(* Logix 5000 AddOnInstructionDefinition export PRNG; software revision 30.00 *)

ADD_ON_INSTRUCTION D_SHR   (* revision 1.0 20170524, vendor Kenneth A. Fischer *)
// DINT bit shift right of the 32-bit argument Inp_A by Inp_B bits with paddding by zeros on the right
// Revision note:
// Rev1.0: 20170524 - Initial Release
VAR_IN_OUT
   Inp_A : DINT; {required}   // 64-bit Integer to be right circular rotated
END_VAR
VAR_INPUT
   Inp_B : INT; {required}   // Number of bits to shift
END_VAR
VAR_IN_OUT
   Out : DINT; {required}   // Result
END_VAR
VAR
   BSR_Cntrl : CONTROL := (LEN := 32);
   ONS : BOOL;
   Source_Bit : BOOL;
   Wrk_InpA : DINT[2];
END_VAR

ROUTINE Logic   (* ladder *)
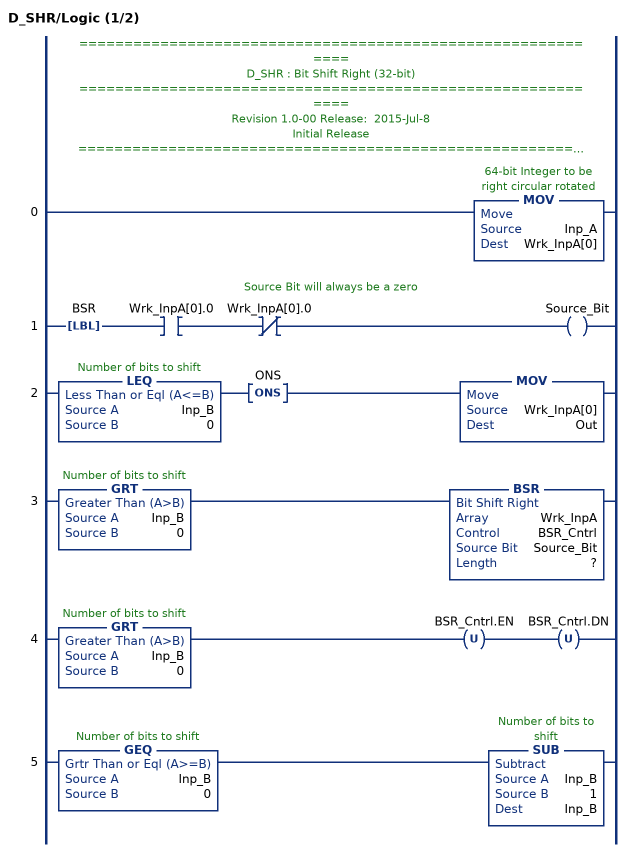
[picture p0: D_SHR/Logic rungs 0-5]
   // ============================================================
   // D_SHR : Bit Shift Right (32-bit)
   // ============================================================
   // Revision 1.0-00 Release:  2015-Jul-8
   // Initial Release
   // ============================================================
   // Performs a right bit shift of the 32-bit argument Inp_A by the
   // number of bits defined in the 16-bit argument Inp_B, with padding by zeros.
   0: MOV(Inp_A,Wrk_InpA[0]);
   // Source Bit will always be a zero
   1: LBL(BSR)XIC(Wrk_InpA[0].0)XIO(Wrk_InpA[0].0)OTE(Source_Bit);
   2: LEQ(Inp_B,0)ONS(ONS)MOV(Wrk_InpA[0],Out);
   3: GRT(Inp_B,0)BSR(Wrk_InpA,BSR_Cntrl,Source_Bit,?);
   4: GRT(Inp_B,0)OTU(BSR_Cntrl.EN)OTU(BSR_Cntrl.DN);
   5: GEQ(Inp_B,0)SUB(Inp_B,1,Inp_B);
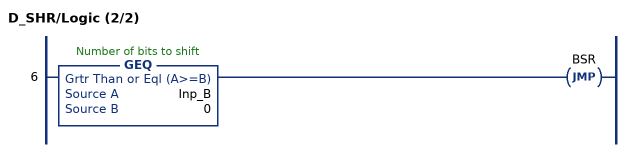
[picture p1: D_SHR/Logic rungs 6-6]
   6: GEQ(Inp_B,0)JMP(BSR);
END_ROUTINE
END_ADD_ON_INSTRUCTION

ADD_ON_INSTRUCTION D_SHL   (* revision 1.0 20170524, vendor Kenneth A. Fischer *)
// DINT bit shift left of the 32-bit argument Inp_A by Inp_B bits with paddding by zeros on the right
// Revision note:
// Rev1.0: 20170524 - Initial Release
VAR_IN_OUT
   Inp_A : DINT; {required}   // 64-bit Integer to be right circular rotated
END_VAR
VAR_INPUT
   Inp_B : INT; {required}   // Number of bits to shift
END_VAR
VAR_IN_OUT
   Out : DINT; {required}   // Result
END_VAR
VAR
   Wrk_InpA : DINT[2];
   Source_Bit : BOOL;
   ONS : BOOL;
   BSL_Cntrl : CONTROL := (LEN := 32);
END_VAR

ROUTINE Logic   (* ladder *)
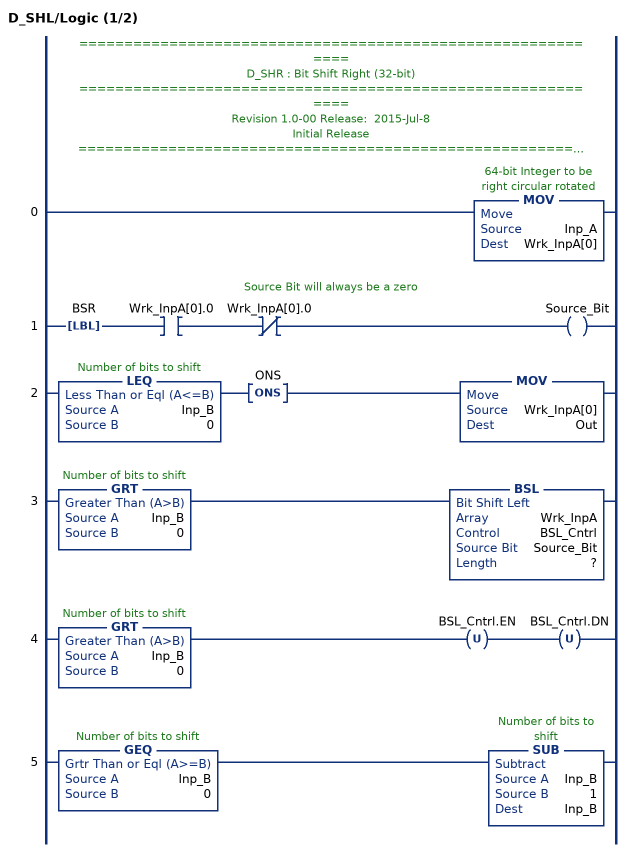
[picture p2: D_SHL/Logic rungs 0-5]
   // ============================================================
   // D_SHR : Bit Shift Right (32-bit)
   // ============================================================
   // Revision 1.0-00 Release:  2015-Jul-8
   // Initial Release
   // ============================================================
   // Performs a left bit shift of the 32-bit argument Inp_A by the
   // number of bits defined in the 16-bit argument Inp_B, with padding by zeros.
   0: MOV(Inp_A,Wrk_InpA[0]);
   // Source Bit will always be a zero
   1: LBL(BSR)XIC(Wrk_InpA[0].0)XIO(Wrk_InpA[0].0)OTE(Source_Bit);
   2: LEQ(Inp_B,0)ONS(ONS)MOV(Wrk_InpA[0],Out);
   3: GRT(Inp_B,0)BSL(Wrk_InpA,BSL_Cntrl,Source_Bit,?);
   4: GRT(Inp_B,0)OTU(BSL_Cntrl.EN)OTU(BSL_Cntrl.DN);
   5: GEQ(Inp_B,0)SUB(Inp_B,1,Inp_B);
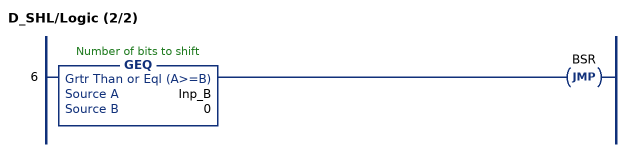
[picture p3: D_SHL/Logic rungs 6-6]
   6: GEQ(Inp_B,0)JMP(BSR);
END_ROUTINE
END_ADD_ON_INSTRUCTION

ADD_ON_INSTRUCTION B256_CtoE   (* revision 1.0 20170916, vendor Kenneth A. Fischer *)
// Convert 256-bit value using 22 12-bit pieces into 256-bit value using 32 8-bit pieces
// Revision note:
// Rev1.0: 20170916 - Initial Release
VAR_IN_OUT
   Inp_C : DINT[22]; {required}
   Out_E : DINT[32]; {required}
END_VAR
VAR
   i : INT;
   j : INT;
   TEMP1 : DINT;
   TEMP2 : DINT;
   D_SHL : D_SHL;
   D_SHR : D_SHR;
END_VAR

ROUTINE Logic   (* ladder *)
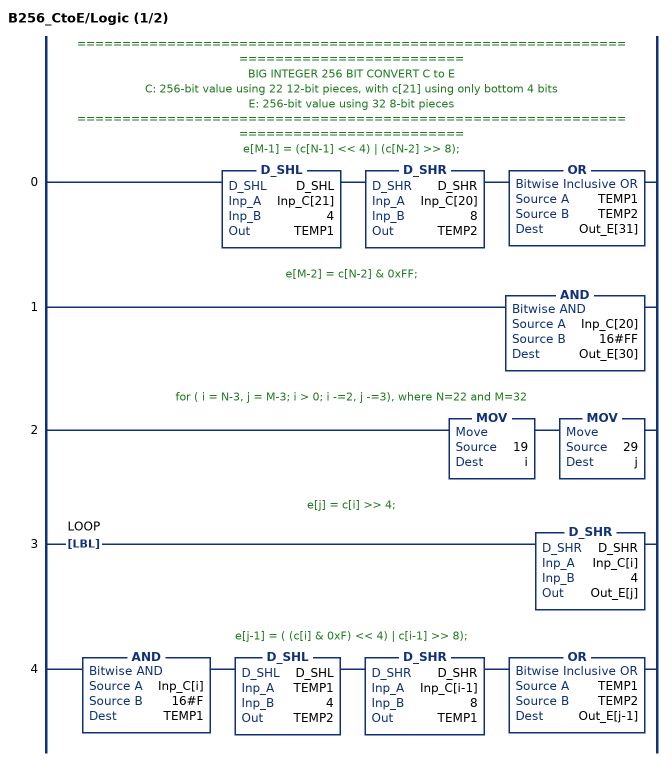
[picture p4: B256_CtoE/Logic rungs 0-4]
   // ======================================================================================
   // BIG INTEGER 256 BIT CONVERT C to E
   // C: 256-bit value using 22 12-bit pieces, with c[21] using only bottom 4 bits
   // E: 256-bit value using 32 8-bit pieces
   // ======================================================================================
   // e[M-1] = (c[N-1] << 4) | (c[N-2] >> 8);
   0: D_SHL(D_SHL,Inp_C[21],4,TEMP1)D_SHR(D_SHR,Inp_C[20],8,TEMP2)OR(TEMP1,TEMP2,Out_E[31]);
   // e[M-2] = c[N-2] & 0xFF;
   1: AND(Inp_C[20],16#FF,Out_E[30]);
   // for ( i = N-3, j = M-3; i > 0; i -=2, j -=3), where N=22 and M=32
   2: MOV(19,i)MOV(29,j);
   // e[j] = c[i] >> 4;
   3: LBL(LOOP)D_SHR(D_SHR,Inp_C[i],4,Out_E[j]);
   // e[j-1] = ( (c[i] & 0xF) << 4) | c[i-1] >> 8);
   4: AND(Inp_C[i],16#F,TEMP1)D_SHL(D_SHL,TEMP1,4,TEMP2)D_SHR(D_SHR,Inp_C[i-1],8,TEMP1)OR(TEMP1,TEMP2,Out_E[j-1]);
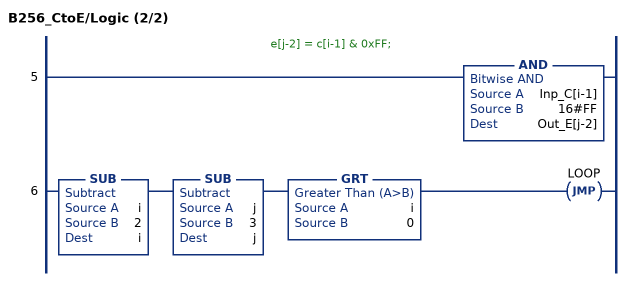
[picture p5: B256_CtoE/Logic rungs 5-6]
   // e[j-2] = c[i-1] & 0xFF;
   5: AND(Inp_C[i-1],16#FF,Out_E[j-2]);
   6: SUB(i,2,i)SUB(j,3,j)GRT(i,0)JMP(LOOP);
END_ROUTINE
END_ADD_ON_INSTRUCTION

ADD_ON_INSTRUCTION B256_CtoS   (* revision 1.0 20170916, vendor Kenneth A. Fischer *)
// Convert 256-bit value using 22 12-bit pieces into 64 hex big endian string characters
// Revision note:
// Rev1.0: 20170916 - Initial Release
VAR_IN_OUT
   Inp_C : DINT[22]; {required}
   Out_S : STRING; {required}
END_VAR
VAR
   byte : DINT[3];
   i : INT;
   j : INT;
   k : DINT;
   D_SHR : D_SHR;
END_VAR

ROUTINE Logic   (* ladder *)
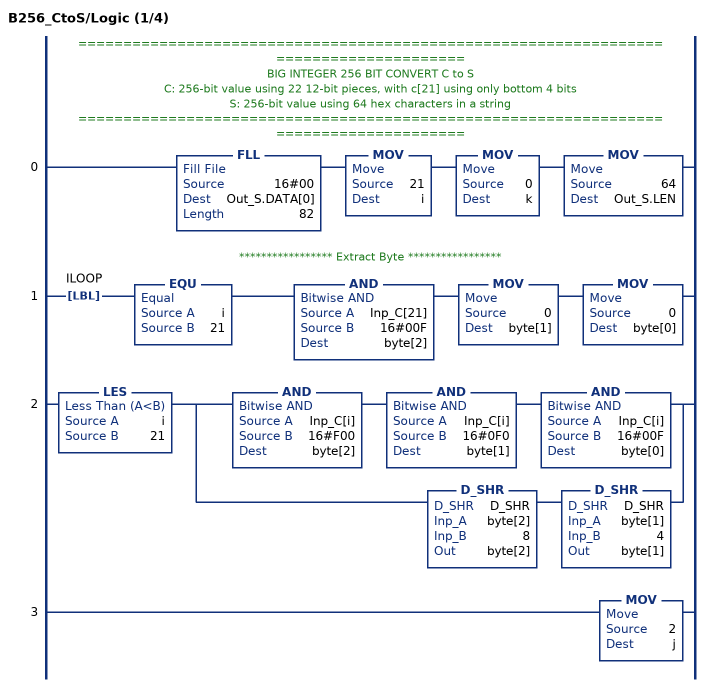
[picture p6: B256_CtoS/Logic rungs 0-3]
   // ======================================================================================
   // BIG INTEGER 256 BIT CONVERT C to S
   // C: 256-bit value using 22 12-bit pieces, with c[21] using only bottom 4 bits
   // S: 256-bit value using 64 hex characters in a string
   // ======================================================================================
   0: FLL(16#00,Out_S.DATA[0],82)MOV(21,i)MOV(0,k)MOV(64,Out_S.LEN);
   // ***************** Extract Byte *****************
   1: LBL(ILOOP)EQU(i,21)AND(Inp_C[21],16#00F,byte[2])MOV(0,byte[1])MOV(0,byte[0]);
   2: LES(i,21)[AND(Inp_C[i],16#F00,byte[2]) AND(Inp_C[i],16#0F0,byte[1]) AND(Inp_C[i],16#00F,byte[0]) ,D_SHR(D_SHR,byte[2],8,byte[2]) D_SHR(D_SHR,byte[1],4,byte[1]) ];
   3: MOV(2,j);
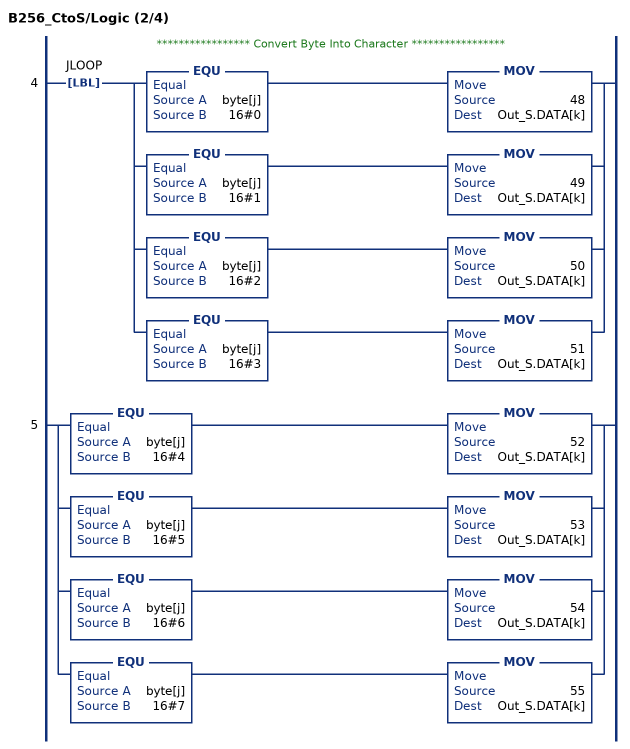
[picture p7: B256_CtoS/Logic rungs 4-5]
   // ***************** Convert Byte Into Character *****************
   4: LBL(JLOOP)[EQU(byte[j],16#0) MOV(48,Out_S.DATA[k]) ,EQU(byte[j],16#1) MOV(49,Out_S.DATA[k]) ,EQU(byte[j],16#2) MOV(50,Out_S.DATA[k]) ,EQU(byte[j],16#3) MOV(51,Out_S.DATA[k]) ];
   5: [EQU(byte[j],16#4) MOV(52,Out_S.DATA[k]) ,EQU(byte[j],16#5) MOV(53,Out_S.DATA[k]) ,EQU(byte[j],16#6) MOV(54,Out_S.DATA[k]) ,EQU(byte[j],16#7) MOV(55,Out_S.DATA[k]) ];
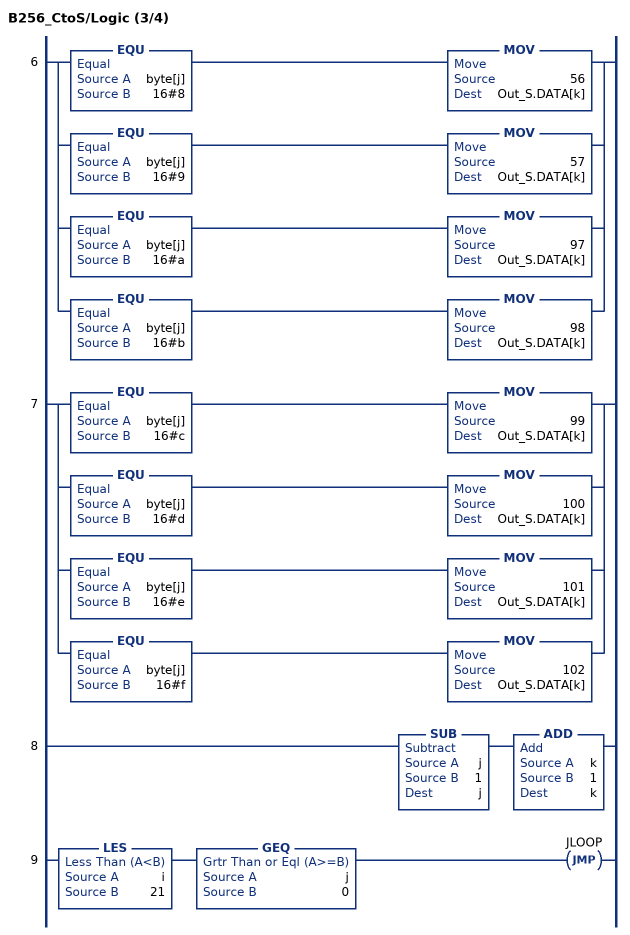
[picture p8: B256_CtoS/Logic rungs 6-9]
   6: [EQU(byte[j],16#8) MOV(56,Out_S.DATA[k]) ,EQU(byte[j],16#9) MOV(57,Out_S.DATA[k]) ,EQU(byte[j],16#a) MOV(97,Out_S.DATA[k]) ,EQU(byte[j],16#b) MOV(98,Out_S.DATA[k]) ];
   7: [EQU(byte[j],16#c) MOV(99,Out_S.DATA[k]) ,EQU(byte[j],16#d) MOV(100,Out_S.DATA[k]) ,EQU(byte[j],16#e) MOV(101,Out_S.DATA[k]) ,EQU(byte[j],16#f) MOV(102,Out_S.DATA[k]) ];
   8: SUB(j,1,j)ADD(k,1,k);
   9: LES(i,21)GEQ(j,0)JMP(JLOOP);
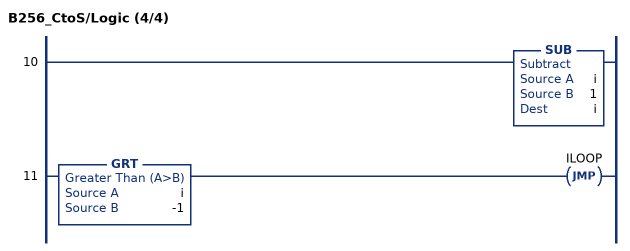
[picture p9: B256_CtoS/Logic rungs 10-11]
   10: SUB(i,1,i);
   11: GRT(i,-1)JMP(ILOOP);
END_ROUTINE
END_ADD_ON_INSTRUCTION

ADD_ON_INSTRUCTION B256_EtoL   (* revision 1.0 20170916, vendor Kenneth A. Fischer *)
// Convert 256-bit value using 32 8-bit pieces into 256-bit value using 4 64-bit pieces
// Revision note:
// Rev1.0: 20170916 - Initial Release
VAR_IN_OUT
   Inp_E : DINT[32]; {required}
   Out_L : LINT[4]; {required}
END_VAR
VAR
   D_SHL : D_SHL;
   Wrk_Out : DINT[2];
   i : INT;
   j : INT;
   TEMP : DINT;
END_VAR

ROUTINE Logic   (* ladder *)
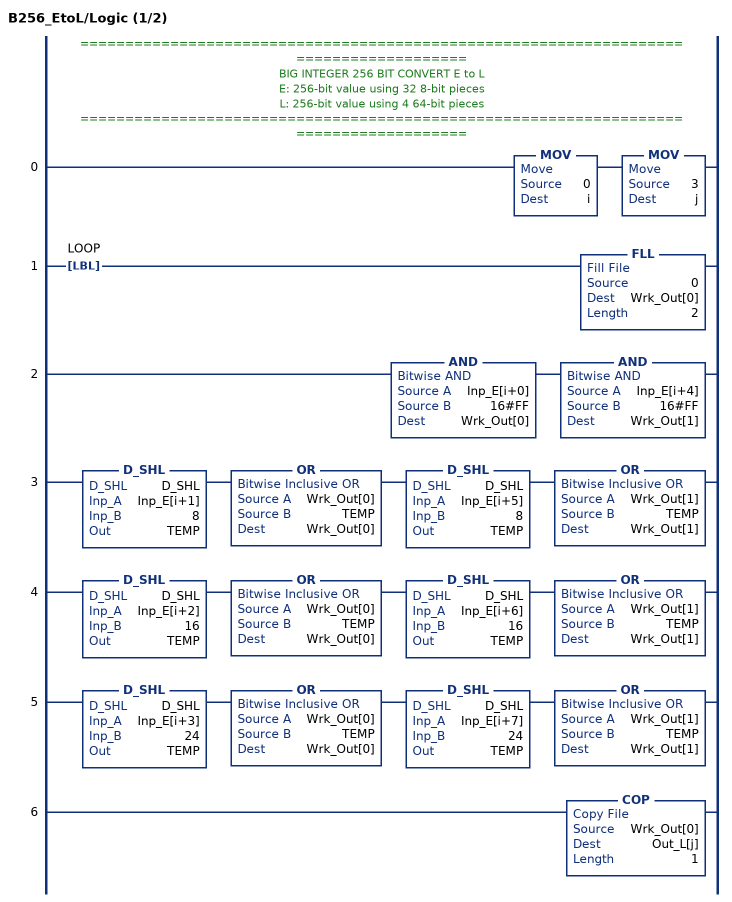
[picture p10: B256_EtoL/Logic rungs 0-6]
   // ======================================================================================
   // BIG INTEGER 256 BIT CONVERT E to L
   // E: 256-bit value using 32 8-bit pieces
   // L: 256-bit value using 4 64-bit pieces
   // ======================================================================================
   0: MOV(0,i)MOV(3,j);
   1: LBL(LOOP)FLL(0,Wrk_Out[0],2);
   2: AND(Inp_E[i+0],16#FF,Wrk_Out[0])AND(Inp_E[i+4],16#FF,Wrk_Out[1]);
   3: D_SHL(D_SHL,Inp_E[i+1],8,TEMP)OR(Wrk_Out[0],TEMP,Wrk_Out[0])D_SHL(D_SHL,Inp_E[i+5],8,TEMP)OR(Wrk_Out[1],TEMP,Wrk_Out[1]);
   4: D_SHL(D_SHL,Inp_E[i+2],16,TEMP)OR(Wrk_Out[0],TEMP,Wrk_Out[0])D_SHL(D_SHL,Inp_E[i+6],16,TEMP)OR(Wrk_Out[1],TEMP,Wrk_Out[1]);
   5: D_SHL(D_SHL,Inp_E[i+3],24,TEMP)OR(Wrk_Out[0],TEMP,Wrk_Out[0])D_SHL(D_SHL,Inp_E[i+7],24,TEMP)OR(Wrk_Out[1],TEMP,Wrk_Out[1]);
   6: COP(Wrk_Out[0],Out_L[j],1);
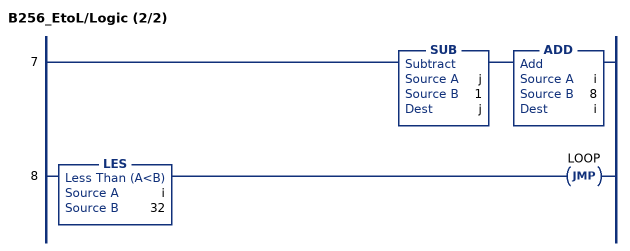
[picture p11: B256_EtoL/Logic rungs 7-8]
   7: SUB(j,1,j)ADD(i,8,i);
   8: LES(i,32)JMP(LOOP);
END_ROUTINE
END_ADD_ON_INSTRUCTION

ADD_ON_INSTRUCTION B256_StoC   (* revision 1.0 20170916, vendor Kenneth A. Fischer *)
// Convert 256-bit value using 64 hex string characters into 256-bit value using 22 12-bit pieces
// Revision note:
// Rev1.0: 20170916 - Initial Release
VAR_IN_OUT
   Inp_S : STRING; {required}
   Out_C : DINT[22]; {required}
END_VAR
VAR
   byte : DINT[3];
   D_SHL : D_SHL;
   i : INT;
   j : INT;
   k : DINT;
   temp : DINT;
END_VAR

ROUTINE Logic   (* ladder *)
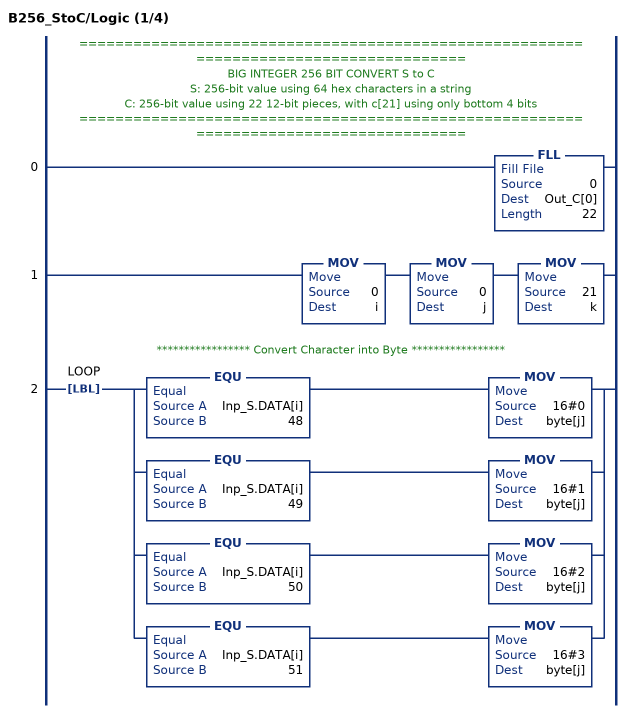
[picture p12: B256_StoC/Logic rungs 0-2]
   // ======================================================================================
   // BIG INTEGER 256 BIT CONVERT S to C
   // S: 256-bit value using 64 hex characters in a string
   // C: 256-bit value using 22 12-bit pieces, with c[21] using only bottom 4 bits
   // ======================================================================================
   0: FLL(0,Out_C[0],22);
   1: MOV(0,i)MOV(0,j)MOV(21,k);
   // ***************** Convert Character into Byte *****************
   2: LBL(LOOP)[EQU(Inp_S.DATA[i],48) MOV(16#0,byte[j]) ,EQU(Inp_S.DATA[i],49) MOV(16#1,byte[j]) ,EQU(Inp_S.DATA[i],50) MOV(16#2,byte[j]) ,EQU(Inp_S.DATA[i],51) MOV(16#3,byte[j]) ];
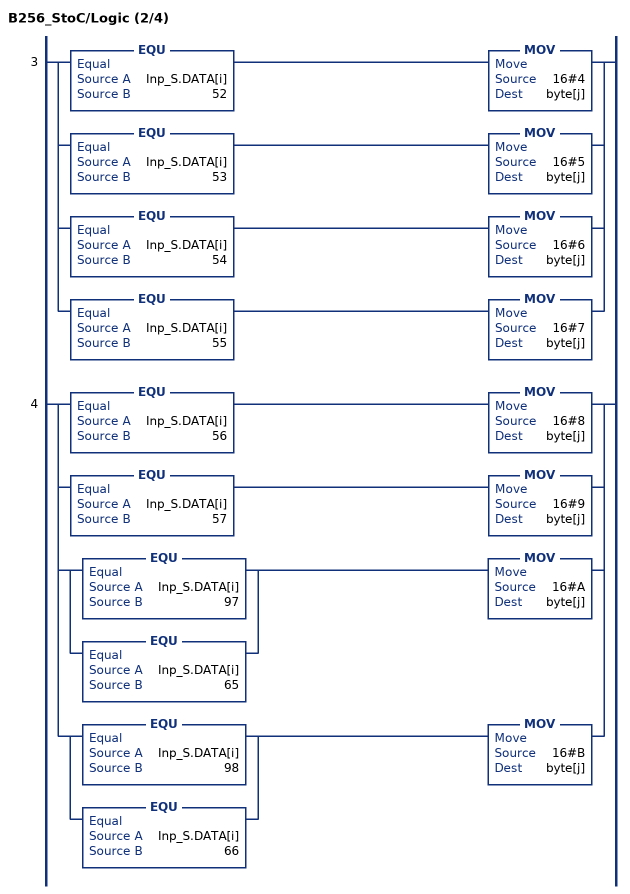
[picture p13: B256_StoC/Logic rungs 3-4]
   3: [EQU(Inp_S.DATA[i],52) MOV(16#4,byte[j]) ,EQU(Inp_S.DATA[i],53) MOV(16#5,byte[j]) ,EQU(Inp_S.DATA[i],54) MOV(16#6,byte[j]) ,EQU(Inp_S.DATA[i],55) MOV(16#7,byte[j]) ];
   4: [EQU(Inp_S.DATA[i],56) MOV(16#8,byte[j]) ,EQU(Inp_S.DATA[i],57) MOV(16#9,byte[j]) ,[EQU(Inp_S.DATA[i],97) ,EQU(Inp_S.DATA[i],65) ] MOV(16#A,byte[j]) ,[EQU(Inp_S.DATA[i],98) ,EQU(Inp_S.DATA[i],66) ] MOV(16#B,byte[j]) ];
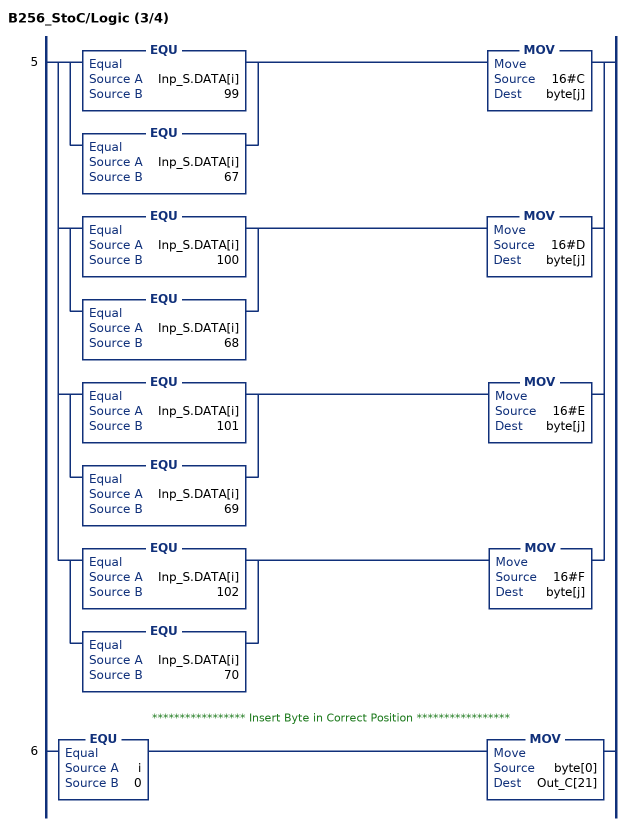
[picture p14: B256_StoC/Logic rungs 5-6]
   5: [[EQU(Inp_S.DATA[i],99) ,EQU(Inp_S.DATA[i],67) ] MOV(16#C,byte[j]) ,[EQU(Inp_S.DATA[i],100) ,EQU(Inp_S.DATA[i],68) ] MOV(16#D,byte[j]) ,[EQU(Inp_S.DATA[i],101) ,EQU(Inp_S.DATA[i],69) ] MOV(16#E,byte[j]) ,[EQU(Inp_S.DATA[i],102) ,EQU(Inp_S.DATA[i],70) ] MOV(16#F,byte[j]) ];
   // ***************** Insert Byte in Correct Position *****************
   6: EQU(i,0)MOV(byte[0],Out_C[21]);
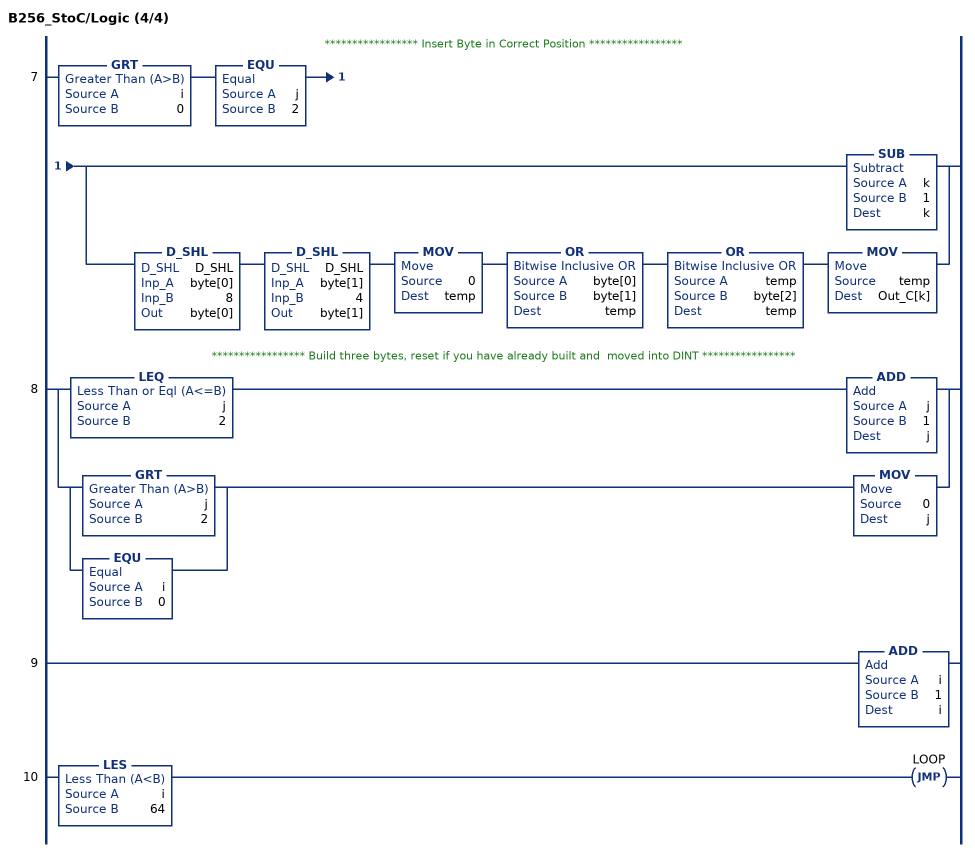
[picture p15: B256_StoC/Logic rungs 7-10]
   // ***************** Insert Byte in Correct Position *****************
   7: GRT(i,0)EQU(j,2)[SUB(k,1,k) ,D_SHL(D_SHL,byte[0],8,byte[0]) D_SHL(D_SHL,byte[1],4,byte[1]) MOV(0,temp) OR(byte[0],byte[1],temp) OR(temp,byte[2],temp) MOV(temp,Out_C[k]) ];
   // ***************** Build three bytes, reset if you have already built and  moved into DINT *****************
   8: [LEQ(j,2) ADD(j,1,j) ,[GRT(j,2) ,EQU(i,0) ] MOV(0,j) ];
   9: ADD(i,1,i);
   10: LES(i,64)JMP(LOOP);
END_ROUTINE
END_ADD_ON_INSTRUCTION

ADD_ON_INSTRUCTION B512_HtoD   (* revision 1.0 20170916, vendor Kenneth A. Fischer *)
// Takes a 512-bit hash value stored as 8 64-bit pieces and converts it to a 512-bit value stored as 42 12-bit pieces and 1 8-bit piece as the MSB
// Revision note:
// Rev1.0: 20170916 - Initial Release
VAR_IN_OUT
   Inp_H : LINT[8]; {required}
   Out_D : DINT[43]; {required}
END_VAR
VAR
   i : INT := 41;
   j : INT := 62;
   Wrk_InpL : DINT[16];
   D_SHR : D_SHR;
   TEMP1 : DINT;
   D_SHL : D_SHL;
   TEMP2 : DINT;
   EE : DINT[64];
END_VAR

ROUTINE Logic   (* ladder *)
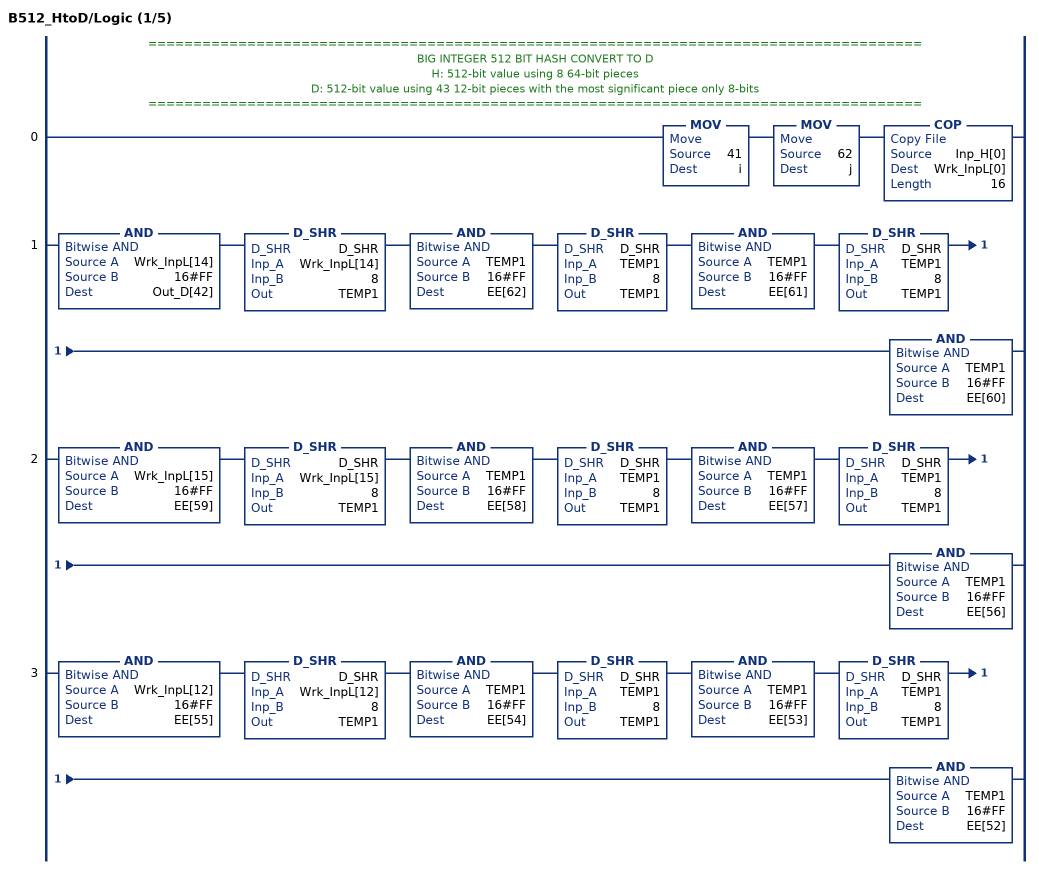
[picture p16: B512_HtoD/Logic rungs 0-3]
   // ======================================================================================
   // BIG INTEGER 512 BIT HASH CONVERT TO D
   // H: 512-bit value using 8 64-bit pieces
   // D: 512-bit value using 43 12-bit pieces with the most significant piece only 8-bits
   // ======================================================================================
   0: MOV(41,i)MOV(62,j)COP(Inp_H[0],Wrk_InpL[0],16);
   1: AND(Wrk_InpL[14],16#FF,Out_D[42])D_SHR(D_SHR,Wrk_InpL[14],8,TEMP1)AND(TEMP1,16#FF,EE[62])D_SHR(D_SHR,TEMP1,8,TEMP1)AND(TEMP1,16#FF,EE[61])D_SHR(D_SHR,TEMP1,8,TEMP1)AND(TEMP1,16#FF,EE[60]);
   2: AND(Wrk_InpL[15],16#FF,EE[59])D_SHR(D_SHR,Wrk_InpL[15],8,TEMP1)AND(TEMP1,16#FF,EE[58])D_SHR(D_SHR,TEMP1,8,TEMP1)AND(TEMP1,16#FF,EE[57])D_SHR(D_SHR,TEMP1,8,TEMP1)AND(TEMP1,16#FF,EE[56]);
   3: AND(Wrk_InpL[12],16#FF,EE[55])D_SHR(D_SHR,Wrk_InpL[12],8,TEMP1)AND(TEMP1,16#FF,EE[54])D_SHR(D_SHR,TEMP1,8,TEMP1)AND(TEMP1,16#FF,EE[53])D_SHR(D_SHR,TEMP1,8,TEMP1)AND(TEMP1,16#FF,EE[52]);
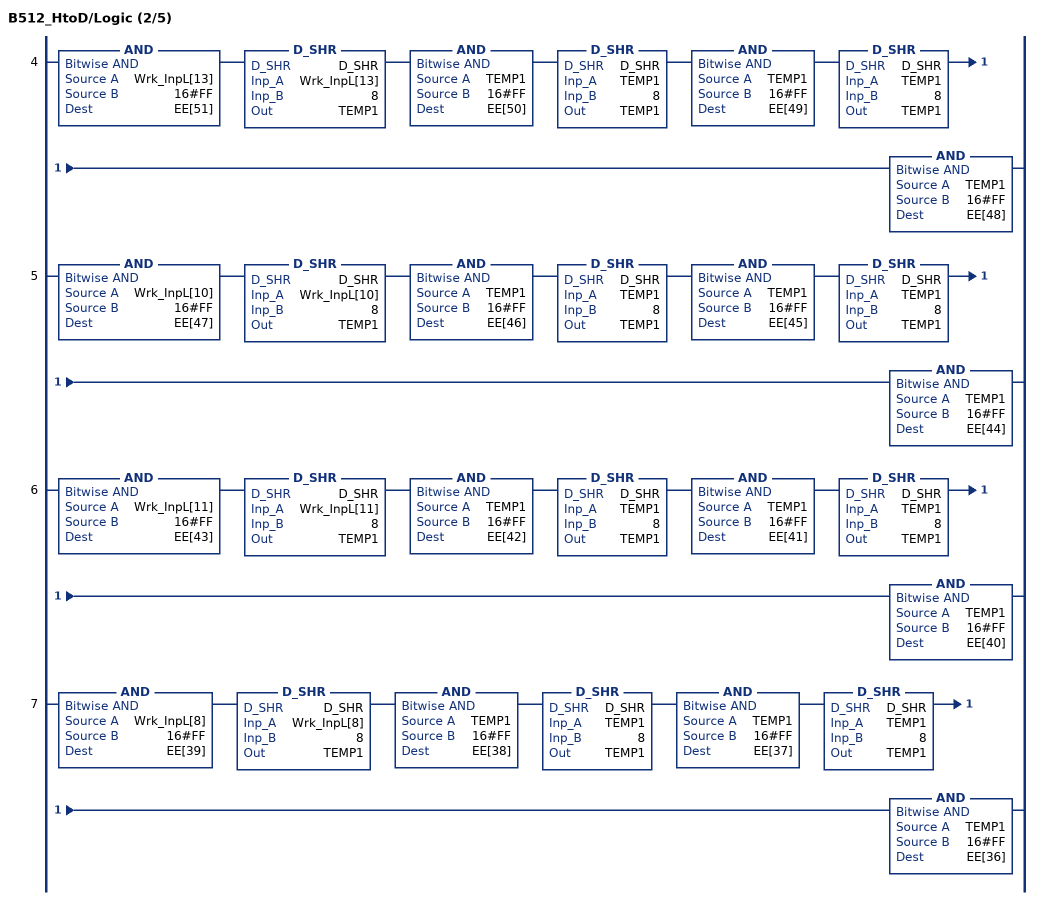
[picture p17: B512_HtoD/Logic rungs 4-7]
   4: AND(Wrk_InpL[13],16#FF,EE[51])D_SHR(D_SHR,Wrk_InpL[13],8,TEMP1)AND(TEMP1,16#FF,EE[50])D_SHR(D_SHR,TEMP1,8,TEMP1)AND(TEMP1,16#FF,EE[49])D_SHR(D_SHR,TEMP1,8,TEMP1)AND(TEMP1,16#FF,EE[48]);
   5: AND(Wrk_InpL[10],16#FF,EE[47])D_SHR(D_SHR,Wrk_InpL[10],8,TEMP1)AND(TEMP1,16#FF,EE[46])D_SHR(D_SHR,TEMP1,8,TEMP1)AND(TEMP1,16#FF,EE[45])D_SHR(D_SHR,TEMP1,8,TEMP1)AND(TEMP1,16#FF,EE[44]);
   6: AND(Wrk_InpL[11],16#FF,EE[43])D_SHR(D_SHR,Wrk_InpL[11],8,TEMP1)AND(TEMP1,16#FF,EE[42])D_SHR(D_SHR,TEMP1,8,TEMP1)AND(TEMP1,16#FF,EE[41])D_SHR(D_SHR,TEMP1,8,TEMP1)AND(TEMP1,16#FF,EE[40]);
   7: AND(Wrk_InpL[8],16#FF,EE[39])D_SHR(D_SHR,Wrk_InpL[8],8,TEMP1)AND(TEMP1,16#FF,EE[38])D_SHR(D_SHR,TEMP1,8,TEMP1)AND(TEMP1,16#FF,EE[37])D_SHR(D_SHR,TEMP1,8,TEMP1)AND(TEMP1,16#FF,EE[36]);
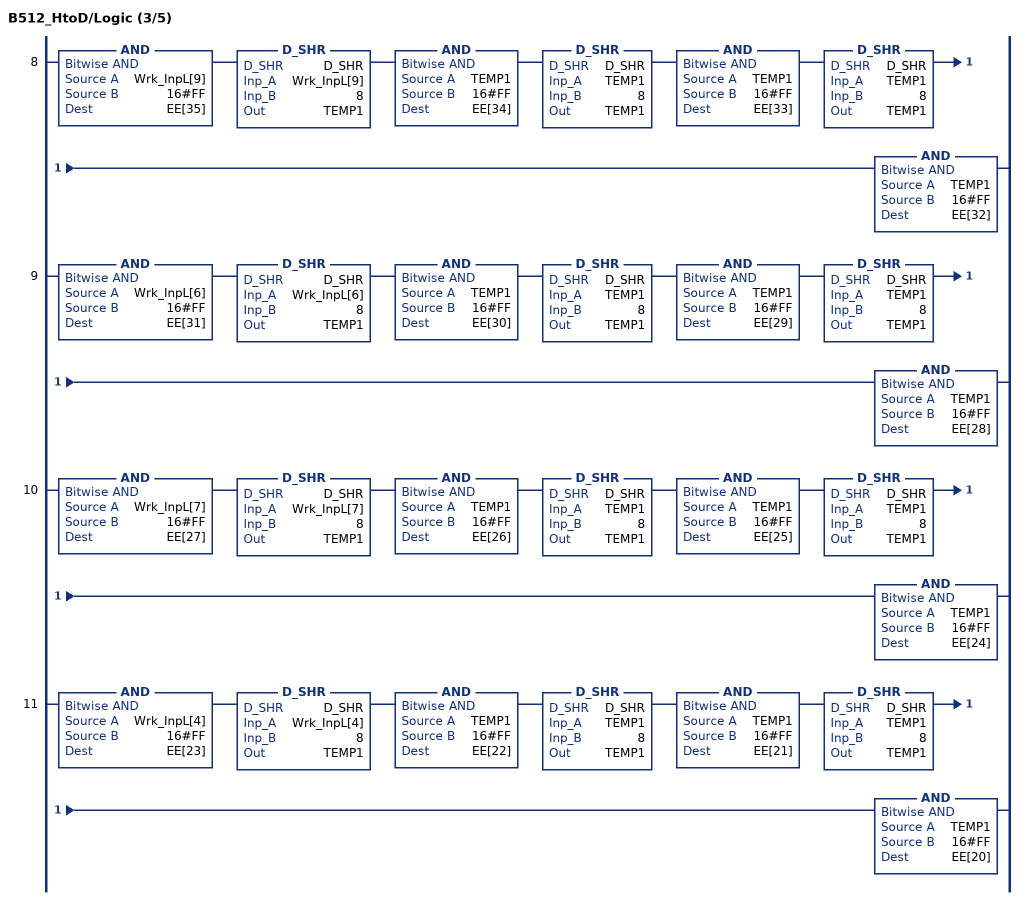
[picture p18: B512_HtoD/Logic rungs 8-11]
   8: AND(Wrk_InpL[9],16#FF,EE[35])D_SHR(D_SHR,Wrk_InpL[9],8,TEMP1)AND(TEMP1,16#FF,EE[34])D_SHR(D_SHR,TEMP1,8,TEMP1)AND(TEMP1,16#FF,EE[33])D_SHR(D_SHR,TEMP1,8,TEMP1)AND(TEMP1,16#FF,EE[32]);
   9: AND(Wrk_InpL[6],16#FF,EE[31])D_SHR(D_SHR,Wrk_InpL[6],8,TEMP1)AND(TEMP1,16#FF,EE[30])D_SHR(D_SHR,TEMP1,8,TEMP1)AND(TEMP1,16#FF,EE[29])D_SHR(D_SHR,TEMP1,8,TEMP1)AND(TEMP1,16#FF,EE[28]);
   10: AND(Wrk_InpL[7],16#FF,EE[27])D_SHR(D_SHR,Wrk_InpL[7],8,TEMP1)AND(TEMP1,16#FF,EE[26])D_SHR(D_SHR,TEMP1,8,TEMP1)AND(TEMP1,16#FF,EE[25])D_SHR(D_SHR,TEMP1,8,TEMP1)AND(TEMP1,16#FF,EE[24]);
   11: AND(Wrk_InpL[4],16#FF,EE[23])D_SHR(D_SHR,Wrk_InpL[4],8,TEMP1)AND(TEMP1,16#FF,EE[22])D_SHR(D_SHR,TEMP1,8,TEMP1)AND(TEMP1,16#FF,EE[21])D_SHR(D_SHR,TEMP1,8,TEMP1)AND(TEMP1,16#FF,EE[20]);
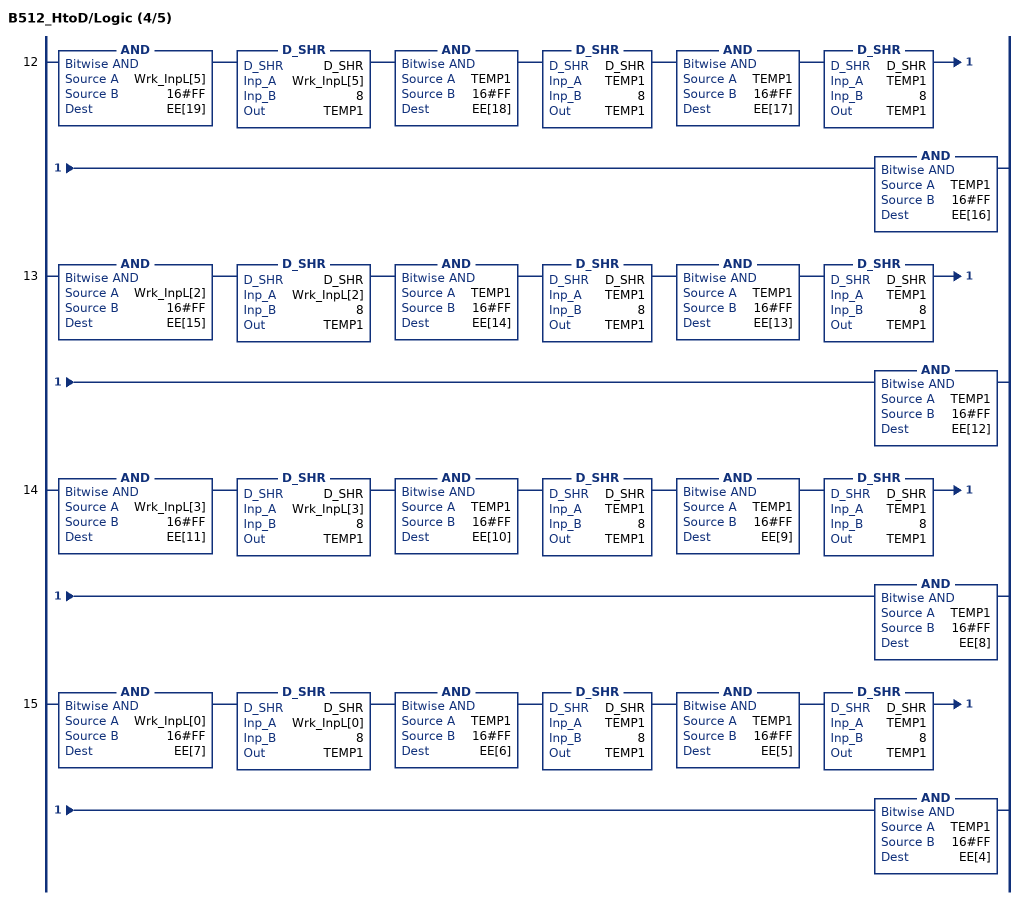
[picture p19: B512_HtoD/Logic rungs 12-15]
   12: AND(Wrk_InpL[5],16#FF,EE[19])D_SHR(D_SHR,Wrk_InpL[5],8,TEMP1)AND(TEMP1,16#FF,EE[18])D_SHR(D_SHR,TEMP1,8,TEMP1)AND(TEMP1,16#FF,EE[17])D_SHR(D_SHR,TEMP1,8,TEMP1)AND(TEMP1,16#FF,EE[16]);
   13: AND(Wrk_InpL[2],16#FF,EE[15])D_SHR(D_SHR,Wrk_InpL[2],8,TEMP1)AND(TEMP1,16#FF,EE[14])D_SHR(D_SHR,TEMP1,8,TEMP1)AND(TEMP1,16#FF,EE[13])D_SHR(D_SHR,TEMP1,8,TEMP1)AND(TEMP1,16#FF,EE[12]);
   14: AND(Wrk_InpL[3],16#FF,EE[11])D_SHR(D_SHR,Wrk_InpL[3],8,TEMP1)AND(TEMP1,16#FF,EE[10])D_SHR(D_SHR,TEMP1,8,TEMP1)AND(TEMP1,16#FF,EE[9])D_SHR(D_SHR,TEMP1,8,TEMP1)AND(TEMP1,16#FF,EE[8]);
   15: AND(Wrk_InpL[0],16#FF,EE[7])D_SHR(D_SHR,Wrk_InpL[0],8,TEMP1)AND(TEMP1,16#FF,EE[6])D_SHR(D_SHR,TEMP1,8,TEMP1)AND(TEMP1,16#FF,EE[5])D_SHR(D_SHR,TEMP1,8,TEMP1)AND(TEMP1,16#FF,EE[4]);
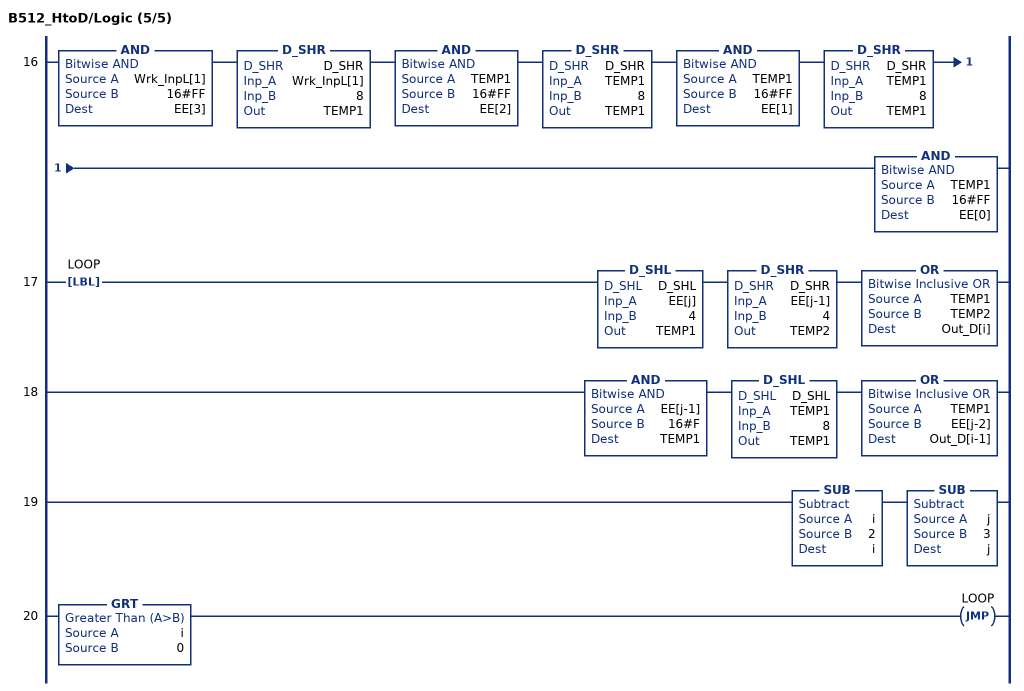
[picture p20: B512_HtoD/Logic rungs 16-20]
   16: AND(Wrk_InpL[1],16#FF,EE[3])D_SHR(D_SHR,Wrk_InpL[1],8,TEMP1)AND(TEMP1,16#FF,EE[2])D_SHR(D_SHR,TEMP1,8,TEMP1)AND(TEMP1,16#FF,EE[1])D_SHR(D_SHR,TEMP1,8,TEMP1)AND(TEMP1,16#FF,EE[0]);
   17: LBL(LOOP)D_SHL(D_SHL,EE[j],4,TEMP1)D_SHR(D_SHR,EE[j-1],4,TEMP2)OR(TEMP1,TEMP2,Out_D[i]);
   18: AND(EE[j-1],16#F,TEMP1)D_SHL(D_SHL,TEMP1,8,TEMP1)OR(TEMP1,EE[j-2],Out_D[i-1]);
   19: SUB(i,2,i)SUB(j,3,j);
   20: GRT(i,0)JMP(LOOP);
END_ROUTINE
END_ADD_ON_INSTRUCTION
